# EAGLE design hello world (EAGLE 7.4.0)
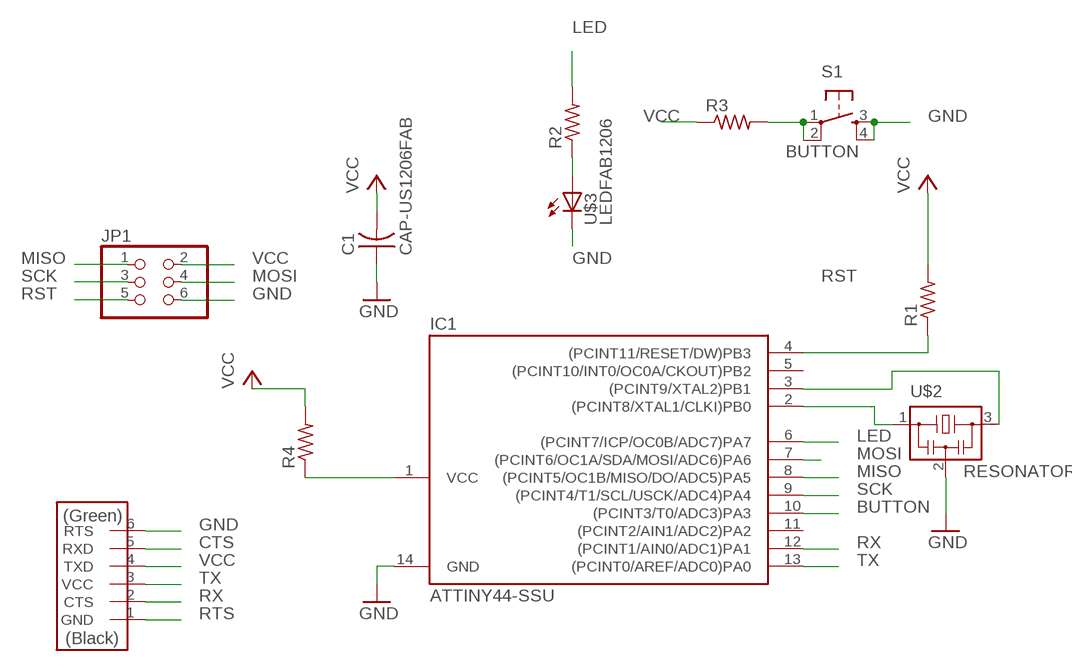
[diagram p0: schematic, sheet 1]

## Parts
C1  CAP-US1206FAB  [C1206FAB]
IC1  ATTINY44-SSU  [SOIC14]
JP1  PINHD-2X3-SMD  [2X03SMD]
R1  RES-US1206FAB  [R1206FAB]
R2  RES-US1206FAB  [R1206FAB]
R3  RES-US1206FAB  [R1206FAB]
R4  RES-US1206FAB  [R1206FAB]
S1  6MM_SWITCH6MM_SWITCH  [6MM_SWITCH]
U$1  FTDI-SMD-HEADER  [1X06SMD]
U$2  RESONATOR  [EFOBM]
U$3  LEDFAB1206  [LED1206FAB]

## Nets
BUTTON: IC1.10((PCINT3/T0/ADC3)PA3) R3.2 S1.1(P) S1.2(P1)
CTS: U$1.5(RXD)
GND: C1.1 IC1.14(GND) JP1.6 S1.3(S) S1.4(S1) U$1.6(RTS) U$2.2 U$3.2(C)
LED: IC1.6((PCINT7/ICP/OC0B/ADC7)PA7) R2.2
MISO: IC1.8((PCINT5/OC1B/MISO/DO/ADC5)PA5) JP1.1
MOSI: IC1.7((PCINT6/OC1A/SDA/MOSI/ADC6)PA6) JP1.4
N$2: IC1.3((PCINT9/XTAL2)PB1) U$2.3
N$3: IC1.2((PCINT8/XTAL1/CLKI)PB0) U$2.1
N$4: R2.1 U$3.1(A)
N$5: IC1.1(VCC) R4.1
RST: IC1.4((PCINT11/RESET/DW)PB3) JP1.5 R1.1
RTS: U$1.1(GND)
RX: IC1.12((PCINT1/AIN0/ADC1)PA1) U$1.2(CTS)
SCK: IC1.9((PCINT4/T1/SCL/USCK/ADC4)PA4) JP1.3
TX: IC1.13((PCINT0/AREF/ADC0)PA0) U$1.3(VCC)
VCC: C1.2 JP1.2 R1.2 R3.1 R4.2 U$1.4(TXD)
Unconnected: IC1.5((PCINT10/INT0/OC0A/CKOUT)PB2) IC1.11((PCINT2/AIN1/ADC2)PA2)

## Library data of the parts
C1 = fab:CAP-US
IC1 = fab:ATTINY44
JP1 = fab:PINHD-2X3-SMD: PIN HEADER
R1-R4 = fab:RES-US: Resistor (US Symbol)
S1 = fab:6MM_SWITCH: OMRON SWITCH
U$1 = fab:FTDI-SMD-HEADER
U$2 = fab:RESONATOR
U$3 = fab:LED: LED

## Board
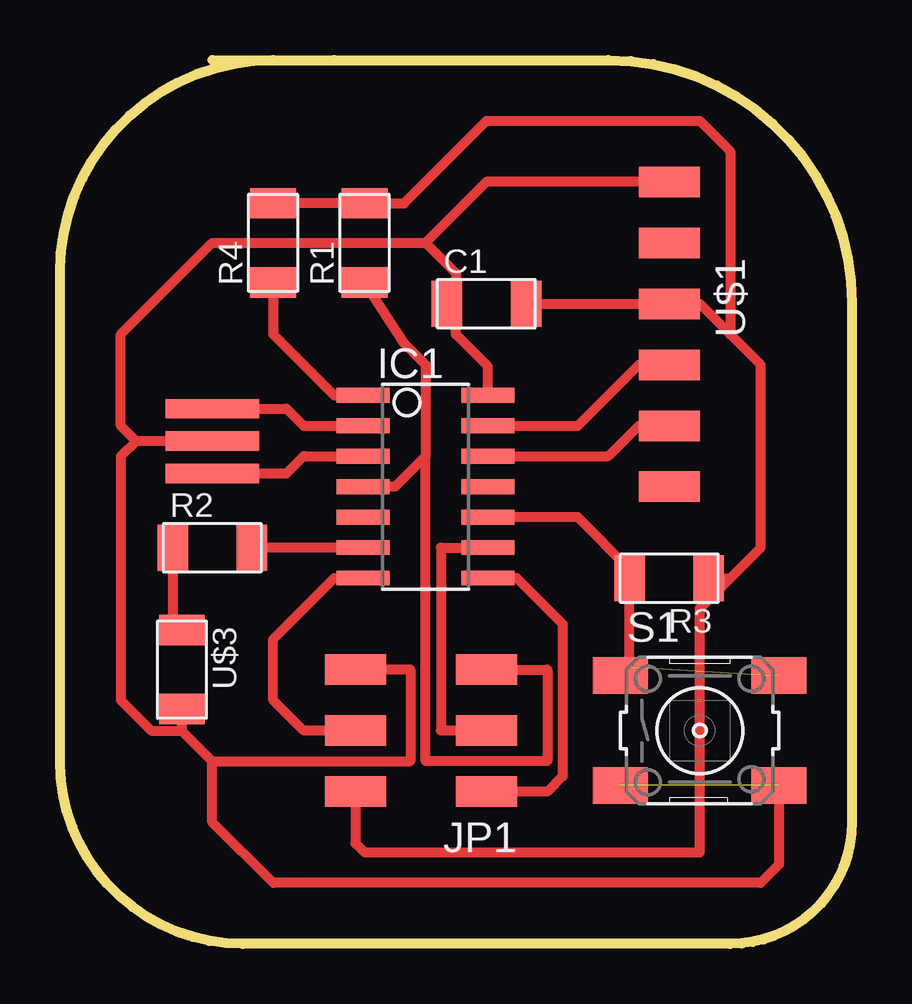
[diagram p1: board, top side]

Size 33.02 x 36.83 mm. Coordinates in mm from the lower left corner, seen from the top.
Outline: 6.35,36.83 8.89,36.83
Outline: 8.89,36.83 arc90 0,27.94 0,7.62 arc90 7.62,0 27.94,0 arc90 33.02,5.08 33.02,26.67 arc90 22.86,36.83 11.43,36.83 8.89,36.83
Copper layers (1*16): Top 0.035mm / dielectric 1.5mm / Bottom 0.035mm
Design rules "default *": minimum track width 10mil, minimum drill 24mil, track to track 16mil, track to pad 16mil, pad to pad 8mil, via to via 8mil, smd to smd 8mil, copper to edge 40mil, drill to drill 8mil, minimum pad ring 10mil, minimum via ring 8mil, stop-mask expansion 4mil, vias tented up to drill 0mil, thermal gap 10mil

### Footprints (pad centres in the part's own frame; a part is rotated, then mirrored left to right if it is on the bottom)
C1206FAB = smd 1.27 x 1.905: 1 -1.651,0; 2 1.651,0
SOIC14 = smd 0.61 x 2.21: 1 -3.81,-2.603; 2 -2.54,-2.603; 3 -1.27,-2.603; 4 0,-2.603; 5 1.27,-2.603; 6 2.54,-2.603; 7 3.81,-2.603; 8 3.81,2.603; 9 2.54,2.603; 10 1.27,2.603; 11 0,2.603; 12 -1.27,2.603; 13 -2.54,2.603; 14 -3.81,2.603
2X03SMD = smd 2.54 x 1.27: 1 -2.54,2.54; 2 2.92,2.54; 3 -2.54,0; 4 2.92,0; 5 -2.54,-2.54; 6 2.92,-2.54
R1206FAB = smd 1.27 x 1.905: 1 -1.651,0; 2 1.651,0
6MM_SWITCH = smd 2.286 x 1.524: 1 -3.302,2.286; 2 3.302,2.286; 3 -3.302,-2.286; 4 3.302,-2.286
1X06SMD = smd 2.54 x 1.27: 1 0,6.35; 2 0,3.81; 3 0,1.27; 4 0,-1.27; 5 0,-3.81; 6 0,-6.35
EFOBM = smd 0.8 x 3.9: 1 -1.35,0; 2 0,0; 3 1.35,0
LED1206FAB = smd 1.27 x 1.905: 1 -1.651,0; 2 1.651,0

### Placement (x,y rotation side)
C1  17.78,26.67 0 top
IC1  15.24,19.05 270 top
JP1  15.24,8.89 180 top
R1  12.7,29.21 90 top
R2  6.35,16.51 0 top
R3  25.4,15.24 180 top
R4  8.89,29.21 90 top
S1  26.67,8.89 0 top
U$1  25.4,25.4 180 top
U$2  6.35,20.95 270 top
U$3  5.08,11.43 270 top

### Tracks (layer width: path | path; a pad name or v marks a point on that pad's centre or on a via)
BUTTON  (1 unrouted)
  Top 0.406: 23.75,11.56 S1.1 23.75,11.18 R3.2 23.75,15.62 21.59,17.78 IC1.10
GND  (1 unrouted)
  Top 0.406: IC1.14 17.84,24.07 16.51,25.4 16.51,26.29 C1.1 16.51,27.05 16.51,27.94 15.24,29.21 | U$3.2 5.08,8.89 | 5.08,8.89 6.35,7.62 | 6.35,7.62 14.6,7.62 14.6,11.43 JP1.6 | S1.4 29.97,3.3 29.21,2.54 8.89,2.54 6.35,5.08 6.35,7.62 | 3.17,20.95 2.54,20.32 2.54,10.16 3.81,8.89 5.08,8.89 | U$2.2 3.17,20.95 | 3.17,20.95 2.54,21.59 2.54,25.4 6.35,29.21 15.24,29.21 | U$1.6 17.78,31.75 15.24,29.21
LED
  Top 0.406: IC1.6 R2.2
MISO
  Top 0.406: IC1.8 19.05,15.24 20.95,13.33 20.95,6.99 20.32,6.35 JP1.1
MOSI
  Top 0.406: 12.7,15.24 IC1.7 11.43,15.24 8.89,12.7 8.89,10.16 10.16,8.89 JP1.4
N$2
  Top 0.406: U$2.3 9.44,19.6 10.16,20.32 IC1.3
N$3
  Top 0.406: U$2.1 9.44,22.3 10.16,21.59 IC1.2
N$4
  Top 0.406: R2.1 4.7,13.46 U$3.1
N$5
  Top 0.406: R4.1 8.89,25.4 11.43,22.86 IC1.1
RST
  Top 0.406: R1.1 14.35,25.02 15.24,24.13 15.24,20.32 | 15.24,20.32 13.97,19.05 IC1.4 | JP1.5 20.32,11.43 20.32,7.62 15.24,7.62 15.24,20.32
RX
  Top 0.406: IC1.12 22.86,20.32 24.13,21.59 U$1.2
SCK
  Top 0.406: JP1.3 15.87,8.89 15.87,16.51 IC1.9
TX
  Top 0.406: IC1.13 21.59,21.59 24.13,24.13 U$1.3
VCC
  Top 0.406: R3.1 27.94,15.24 | 27.94,15.24 29.21,16.51 29.21,24.13 27.94,25.4 | 27.94,25.4 26.67,26.67 U$1.4 C1.2 | JP1.2 12.32,4.19 12.7,3.81 26.67,3.81 26.67,13.97 27.94,15.24 | R4.2 R1.2 14.35,30.86 17.78,34.29 26.67,34.29 27.94,33.02 27.94,25.4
